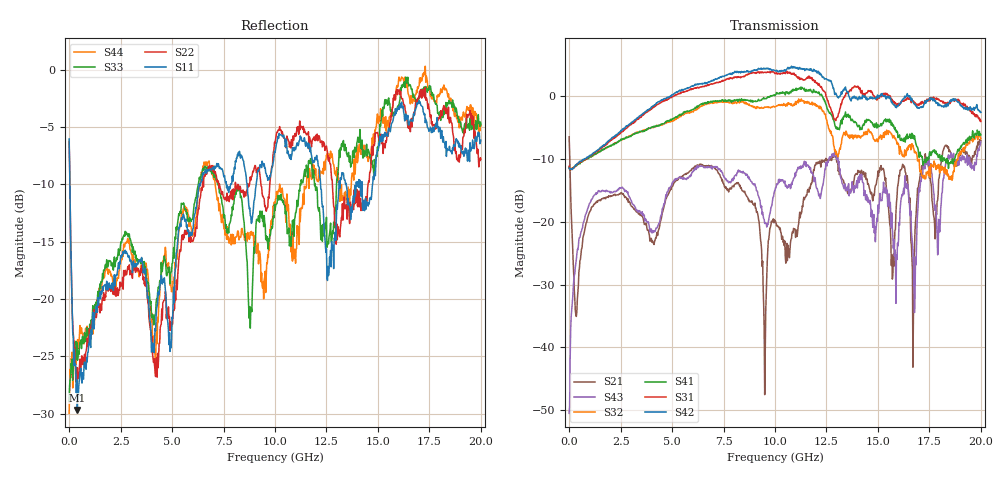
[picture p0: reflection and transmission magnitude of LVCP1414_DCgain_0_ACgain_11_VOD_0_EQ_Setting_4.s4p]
!Agilent Technologies,N5230A,MY46400459,A.07.50.48
!Agilent N5230A: A.07.50.48
!Date: Tuesday, April 17, 2012 18:38:25
!Correction: S11(Full 4 Port(1,2,3,4))
!S12(Full 4 Port(1,2,3,4))
!S13(Full 4 Port(1,2,3,4))
!S14(Full 4 Port(1,2,3,4))
!S21(Full 4 Port(1,2,3,4))
!S22(Full 4 Port(1,2,3,4))
!S23(Full 4 Port(1,2,3,4))
!S24(Full 4 Port(1,2,3,4))
!S31(Full 4 Port(1,2,3,4))
!S32(Full 4 Port(1,2,3,4))
!S33(Full 4 Port(1,2,3,4))
!S34(Full 4 Port(1,2,3,4))
!S41(Full 4 Port(1,2,3,4))
!S42(Full 4 Port(1,2,3,4))
!S43(Full 4 Port(1,2,3,4))
!S44(Full 4 Port(1,2,3,4))
!S4P File: Measurements: <S11,S12,S13,S14>,
!<S21,S22,S23,S24>,
!<S31,S32,S33,S34>,
!<S41,S42,S43,S44>:
# Hz S  dB  R 50
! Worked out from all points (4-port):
!   801 points, 300 kHz to 20 GHz, reference 50 ohm
!   strongest paths, dB at 300 kHz, 5 GHz, 10 GHz, 15 GHz, 20 GHz:
!     S42: -11.5, 0.2, 4.0, 0.1, -2.6
!     S31: -11.2, -0.1, 3.6, -0.4, -4.0
!     S41: -11.3, -3.6, 0.1, -4.5, -6.2
!     S32: -11.4, -4.0, -1.7, -7.3, -6.8
!     S43: -50.5, -13.9, -15.0, -17.3, -7.3
!     S21: -6.5, -14.3, -19.8, -11.9, -7.1
!   lowest |S11| = -29.7 dB at 400.3 MHz (marker M1), VSWR 1.07, Z = 53.1 + j1.48 ohm
!   |S11| at or under -10 dB: 37.62 MHz to 6.323 GHz (6.285 GHz wide, 198 % of centre); 12.21 GHz to 13.11 GHz (900.8 MHz wide, 7.11 % of centre); 14.23 GHz to 14.74 GHz (511.5 MHz wide, 3.53 % of centre)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
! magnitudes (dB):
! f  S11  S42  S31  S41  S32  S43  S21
! 300 kHz  -6.0  -11.5  -11.2  -11.3  -11.4  -50.5  -6.5
! 400.3 MHz  -29.7  -10.8  -10.7  -10.9  -10.8  -24.4  -32.3
! 10.05 GHz  -6.7  4.0  3.6  0.3  -1.6  -14.6  -20.2
! 12.73 GHz  -17.2  2.4  -2.2  -3.0  -5.6  -9.8  -10.0
! 16.78 GHz  -3.8  -1.3  -1.0  -6.3  -9.0  -34.5  -24.6
! 18 GHz  -5.0  -1.5  -0.7  -9.3  -12.2  -21.6  -12.3
! 20 GHz  -6.2  -2.6  -4.0  -6.2  -6.8  -7.3  -7.1
